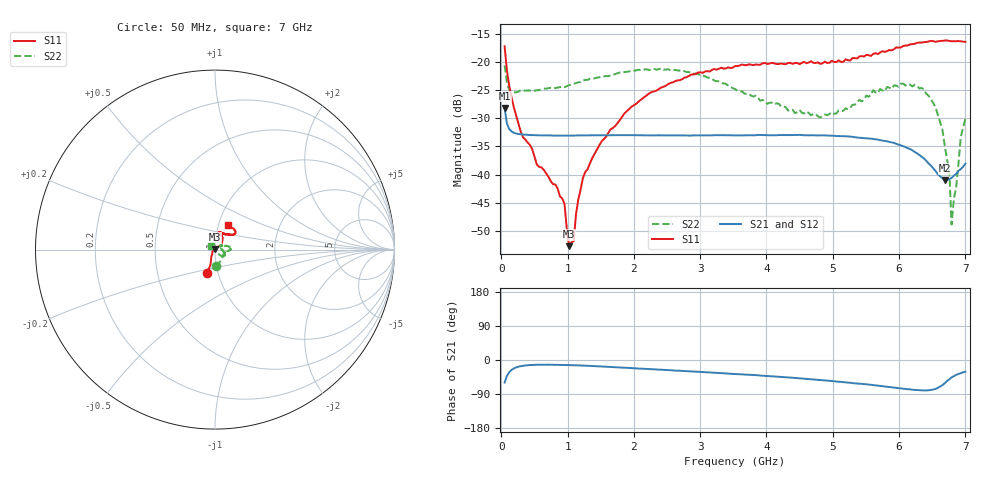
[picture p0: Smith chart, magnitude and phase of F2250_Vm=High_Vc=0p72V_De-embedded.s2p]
! Integrated Device Technology
! Corporate Headquarters
! 6024 Silver Creek Valley Road
! San Jose, CA 95138  USA
! Phone:  1-408-284-8200
! Toll Free:  1-800-223-1366
! Webpage:  http://www.idt.com/
! Timing and RF Division
! 515 Groton Road, Suite 102
! Westford, MA 01886-6024
! Device:  F2250
! Description: Voltage Variable RF Attenuator
! Frequency:  50.0 -  6000.00 MHz
! Package:  3x3 mm Thin QFN Plastic Package: 16 pin
! Ports:  2 RF, 3 DC
!  Pin  1  = GND
!  Pin  2  = NC
!  Pin  3  = RF1  = Port 1
!  Pin  4  = NC
!  Pin  5  = GND
!  Pin  6  = GND
!  Pin  7  = GND
!  Pin  8  = GND
!  Pin  9  = NC
!  Pin 10  = RF2  = Port 2
!  Pin 11  = NC
!  Pin 12  = GND
!  Pin 13  = GND
!  Pin 14  = VCNTRL
!  Pin 15  = VDD
!  Pin 16  = VMODE
! Vcntrl:  0.720 Volts
! Vmode:  +3.300 Volts
! Vdd:  +3.30  Volts
! Current:  1.292 mA
! Data:  The device was measured on a the F2250 evaluation board which has
!  individual transmission lines to the RF pins.  Data was collected
!  using a calibrated network analyzer.  The evaluation board was
!  de-embedded using a TRL calibration technique.
!  The reference plane is the edge of the package pin.
! Misc:  SN 10
!  Action Tracker AT0258
! Date Measured:  2014-11-26
! Date:  2015-10-15  MJV
! Note:
!  Integrated Device Technology supplies this data as a sample of measured
!  data at the package pin for this product.  Your particular data for this
!  product may vary.
!  Data was taken at 25 degrees C.
!  Integrated Device Technology reserves the right to change this data at anytime.
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# GHz S dB R 50
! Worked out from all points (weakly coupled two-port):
!   201 points, 50 MHz to 7 GHz, reference 50 ohm
!   highest |S21| = -28.13 dB at 50 MHz (marker M1); lowest = -41.0 dB at 6.687 GHz (marker M2)
!   lowest |S11| = -52.8 dB at 1.023 GHz (marker M3), VSWR 1.00, Z = 49.8 + j0.161 ohm
!   |S11| at or under -10 dB: start of sweep to end of sweep
!   |S22| runs from -48.9 to -20.6 dB; largest |S21 - S12| = 7.1e-05
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0.05  -17.15 -108.1  -28.13 -59.6  -28.12 -59.6  -20.55 -86.2
0.1195  -24.20 -111.3  -31.89 -32.2  -31.88 -32.1  -24.87 -39.7
0.29325  -32.36 -125.9  -32.83 -16.3  -32.83 -16.2  -24.97 -16.8
0.9535  -45.19 172.2  -33.07 -13.1  -33.06 -13.2  -24.43 -7.9
1.023  -52.75 135.6  -33.06 -13.4  -33.07 -13.4  -24.08 -7.2
1.0925  -51.85 76.3  -33.06 -13.8  -33.05 -13.8  -23.88 -6.9
1.12725  -46.97 53.6  -33.04 -14.0  -33.04 -14.0  -23.68 -7.4
1.2315  -40.61 37.2  -33.03 -14.7  -33.01 -14.7  -23.26 -8.2
1.6485  -31.95 39.8  -32.99 -18.3  -32.98 -18.3  -22.33 -4.6
2.37825  -24.75 46.0  -33.00 -25.3  -33.01 -25.3  -21.21 2.6
3.525  -20.69 71.4  -33.03 -36.8  -33.03 -36.8  -24.77 21.6
4.7065  -20.10 71.8  -33.00 -51.2  -33.00 -51.3  -29.22 25.7
5.054  -19.96 59.9  -33.14 -56.5  -33.13 -56.6  -29.11 9.8
5.85325  -17.82 40.4  -34.18 -71.2  -34.20 -71.3  -24.51 -22.9
6.3745  -16.42 40.8  -37.13 -80.4  -37.13 -80.5  -24.81 -38.8
6.54825  -16.36 44.5  -39.35 -76.3  -39.38 -76.3  -27.99 -49.5
6.68725  -16.13 47.7  -41.01 -61.5  -41.05 -61.1  -34.75 -54.2
6.75675  -16.21 50.4  -40.81 -51.2  -40.80 -51.1  -39.16 -70.5
6.7915  -16.27 51.2  -40.61 -45.9  -40.59 -45.8  -48.89 -87.2
6.861  -16.24 54.3  -39.88 -39.4  -39.87 -39.3  -42.23 178.2
6.9305  -16.26 58.6  -39.02 -34.8  -39.00 -34.9  -33.29 146.6
7  -16.36 62.2  -38.06 -31.0  -38.05 -31.0  -30.02 141.1
